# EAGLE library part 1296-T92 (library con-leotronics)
1.27mm SINGLE ROW FEMALE SOCKET Source: http://www.leotronics.co.uk/Conexcon/Data%20Sheets/sec.%20A/1296ing.pdf
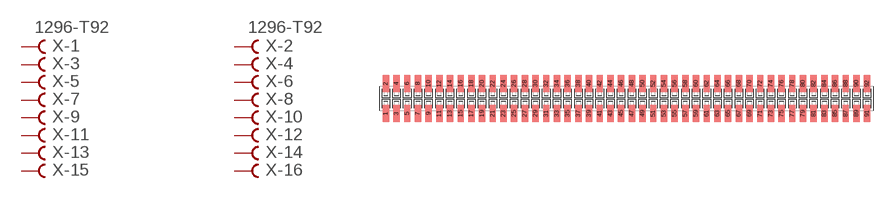
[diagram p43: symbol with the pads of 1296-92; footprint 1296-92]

Designator prefix X; gates -1=FVAL -2=FVAL -3=F -4=F -5=F -6=F -7=F -8=F -9=F -10=F -11=F -12=F -13=F -14=F -15=F -16=F -17=F -18=F -19=F -20=F -21=F -22=F -23=F -24=F -25=F -26=F -27=F -28=F -29=F -30=F -31=F -32=F -33=F -34=F -35=F -36=F -37=F -38=F -39=F -40=F -41=F -42=F -43=F -44=F -45=F -46=F -47=F -48=F -49=F -50=F -51=F -52=F -53=F -54=F -55=F -56=F -57=F -58=F -59=F -60=F -61=F -62=F -63=F -64=F -65=F -66=F -67=F -68=F -69=F -70=F -71=F -72=F -73=F -74=F -75=F -76=F -77=F -78=F -79=F -80=F -81=F -82=F -83=F -84=F -85=F -86=F -87=F -88=F -89=F -90=F -91=F -92=F

## 1296-T92 (OC_FARNELL: unknown; OC_NEWARK: unknown)  [1296-92]
1  -1:B  pas
2  -2:B  pas
3  -3:B  pas
4  -4:B  pas
5  -5:B  pas
6  -6:B  pas
7  -7:B  pas
8  -8:B  pas
9  -9:B  pas
10  -10:B  pas
11  -11:B  pas
12  -12:B  pas
13  -13:B  pas
14  -14:B  pas
15  -15:B  pas
16  -16:B  pas
17  -17:B  pas
18  -18:B  pas
19  -19:B  pas
20  -20:B  pas
21  -21:B  pas
22  -22:B  pas
23  -23:B  pas
24  -24:B  pas
25  -25:B  pas
26  -26:B  pas
27  -27:B  pas
28  -28:B  pas
29  -29:B  pas
30  -30:B  pas
31  -31:B  pas
32  -32:B  pas
33  -33:B  pas
34  -34:B  pas
35  -35:B  pas
36  -36:B  pas
37  -37:B  pas
38  -38:B  pas
39  -39:B  pas
40  -40:B  pas
41  -41:B  pas
42  -42:B  pas
43  -43:B  pas
44  -44:B  pas
45  -45:B  pas
46  -46:B  pas
47  -47:B  pas
48  -48:B  pas
49  -49:B  pas
50  -50:B  pas
51  -51:B  pas
52  -52:B  pas
53  -53:B  pas
54  -54:B  pas
55  -55:B  pas
56  -56:B  pas
57  -57:B  pas
58  -58:B  pas
59  -59:B  pas
60  -60:B  pas
61  -61:B  pas
62  -62:B  pas
63  -63:B  pas
64  -64:B  pas
65  -65:B  pas
66  -66:B  pas
67  -67:B  pas
68  -68:B  pas
69  -69:B  pas
70  -70:B  pas
71  -71:B  pas
72  -72:B  pas
73  -73:B  pas
74  -74:B  pas
75  -75:B  pas
76  -76:B  pas
77  -77:B  pas
78  -78:B  pas
79  -79:B  pas
80  -80:B  pas
81  -81:B  pas
82  -82:B  pas
83  -83:B  pas
84  -84:B  pas
85  -85:B  pas
86  -86:B  pas
87  -87:B  pas
88  -88:B  pas
89  -89:B  pas
90  -90:B  pas
91  -91:B  pas
92  -92:B  pas

## Footprint 1296-92 (pad centres in mm)
1.27mm SINGLE ROW FEMALE SOCKET Source: http://www.leotronics.co.uk/Conexcon/Data%20Sheets/sec.%20A/1296ing.pdf
smd 0.76 x 2.05: 1 -28.575,-1.78; 2 -28.575,1.78; 3 -27.305,-1.78; 4 -27.305,1.78; 5 -26.035,-1.78; 6 -26.035,1.78; 7 -24.765,-1.78; 8 -24.765,1.78; 9 -23.495,-1.78; 10 -23.495,1.78; 11 -22.225,-1.78; 12 -22.225,1.78; 13 -20.955,-1.78; 14 -20.955,1.78; 15 -19.685,-1.78; 16 -19.685,1.78; 17 -18.415,-1.78; 18 -18.415,1.78; 19 -17.145,-1.78; 20 -17.145,1.78; 21 -15.875,-1.78; 22 -15.875,1.78; 23 -14.605,-1.78; 24 -14.605,1.78; 25 -13.335,-1.78; 26 -13.335,1.78; 27 -12.065,-1.78; 28 -12.065,1.78; 29 -10.795,-1.78; 30 -10.795,1.78; 31 -9.525,-1.78; 32 -9.525,1.78; 33 -8.255,-1.78; 34 -8.255,1.78; 35 -6.985,-1.78; 36 -6.985,1.78; 37 -5.715,-1.78; 38 -5.715,1.78; 39 -4.445,-1.78; 40 -4.445,1.78; 41 -3.175,-1.78; 42 -3.175,1.78; 43 -1.905,-1.78; 44 -1.905,1.78; 45 -0.635,-1.78; 46 -0.635,1.78; 47 0.635,-1.78; 48 0.635,1.78; 49 1.905,-1.78; 50 1.905,1.78; 51 3.175,-1.78; 52 3.175,1.78; 53 4.445,-1.78; 54 4.445,1.78; 55 5.715,-1.78; 56 5.715,1.78; 57 6.985,-1.78; 58 6.985,1.78; 59 8.255,-1.78; 60 8.255,1.78; 61 9.525,-1.78; 62 9.525,1.78; 63 10.795,-1.78; 64 10.795,1.78; 65 12.065,-1.78; 66 12.065,1.78; 67 13.335,-1.78; 68 13.335,1.78; 69 14.605,-1.78; 70 14.605,1.78; 71 15.875,-1.78; 72 15.875,1.78; 73 17.145,-1.78; 74 17.145,1.78; 75 18.415,-1.78; 76 18.415,1.78; 77 19.685,-1.78; 78 19.685,1.78; 79 20.955,-1.78; 80 20.955,1.78; 81 22.225,-1.78; 82 22.225,1.78; 83 23.495,-1.78; 84 23.495,1.78; 85 24.765,-1.78; 86 24.765,1.78; 87 26.035,-1.78; 88 26.035,1.78; 89 27.305,-1.78; 90 27.305,1.78; 91 28.575,-1.78; 92 28.575,1.78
